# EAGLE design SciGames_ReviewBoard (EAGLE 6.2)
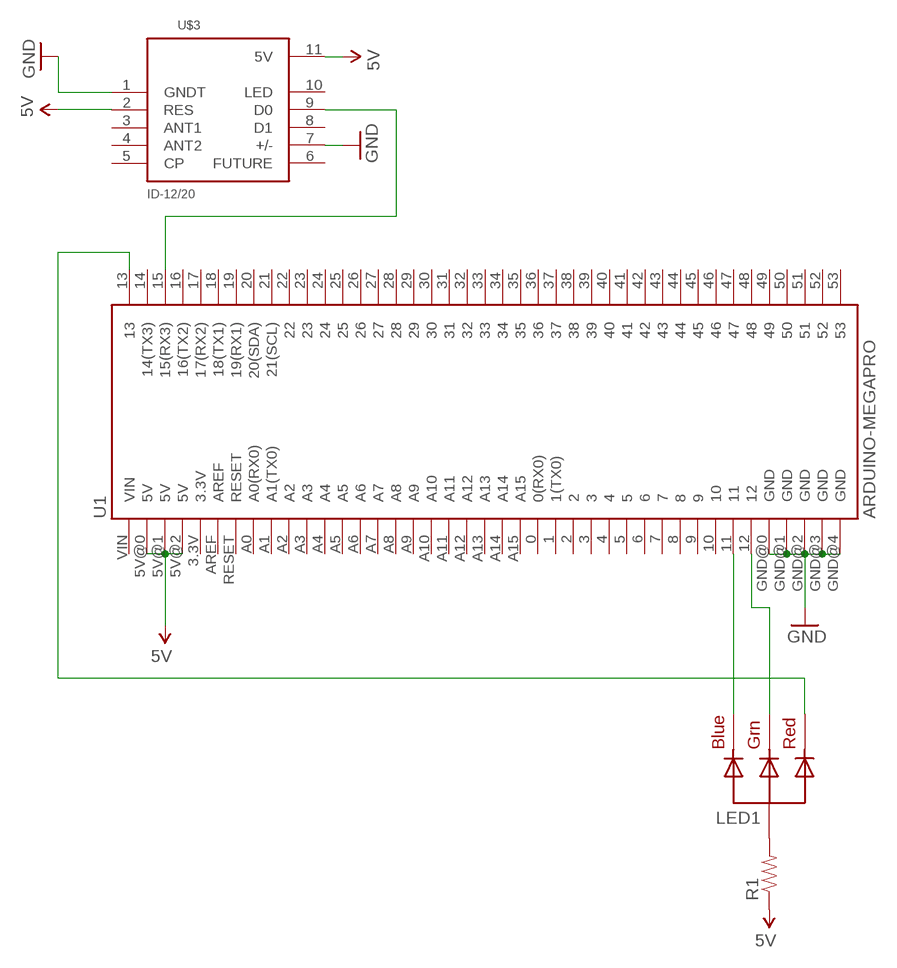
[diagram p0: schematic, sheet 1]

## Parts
LED1  RGBLED_CA-5MM  [LED5MMRGB]
R1  RESISTORPTH-1/6W  [1/6W-RES]
U1  ARDUINO-MEGAPRO  [ARDUINO_MEGA-PRO-3.3V]
U$3  ID-12/20  [ID-12]

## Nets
5V: R1.1 U1.5V@0(5V) U1.5V@1(5V) U1.5V@2(5V) U$3.2(RES) U$3.11(5V)
GND: U1.GND@0(GND) U1.GND@1(GND) U1.GND@2(GND) U1.GND@3(GND) U1.GND@4(GND) U$3.1(GNDT) U$3.7(+/-)
N$1: U1.15(15(RX3)) U$3.9(D0)
N$2: LED1.4(BLUE) U1.11
N$3: LED1.3(GREEN) U1.12
N$4: LED1.1(RED) U1.13
N$5: LED1.2(VCC) R1.2
Unconnected: U1.0(0(RX0)) U1.1(1(TX0)) U1.2 U1.3 U1.3.3V U1.4 U1.5 U1.6 U1.7 U1.8 U1.9 U1.10 U1.14(14(TX3)) U1.16(16(TX2)) U1.17(17(RX2)) U1.18(18(TX1)) U1.19(19(RX1)) U1.20(20(SDA)) U1.21(21(SCL)) U1.22 U1.23 U1.24 U1.25 U1.26 U1.27 U1.28 U1.29 U1.30 U1.31 U1.32 U1.33 U1.34 U1.35 U1.36 U1.37 U1.38 U1.39 U1.40 U1.41 U1.42 U1.43 U1.44 U1.45 U1.46 U1.47 U1.48 U1.49 U1.50 U1.51 U1.52 U1.53 U1.A0(A0(RX0)) U1.A1(A1(TX0)) U1.A2 U1.A3 U1.A4 U1.A5 U1.A6 U1.A7 U1.A8 U1.A9 U1.A10 U1.A11 U1.A12 U1.A13 U1.A14 U1.A15 U1.AREF U1.RESET U1.VIN U$3.3(ANT1) U$3.4(ANT2) U$3.5(CP) U$3.6(FUTURE) U$3.8(D1) U$3.10(LED)

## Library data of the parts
LED1 = adafruit:RGBLED_CA: RGB LED, common-anode 5MM Staggered pins 5mm Piranha package http://www.ladyada.net/library/pcb/eaglelibrary.html
R1 = SparkFun-Passives:RESISTOR: Resistor
U1 = SparkFun:ARDUINO-MEGA: Arduino Mega footprint connections
U$3 = SparkFun-RF:ID-12/20: RFID reader for ID2, ID12, and ID20 Package

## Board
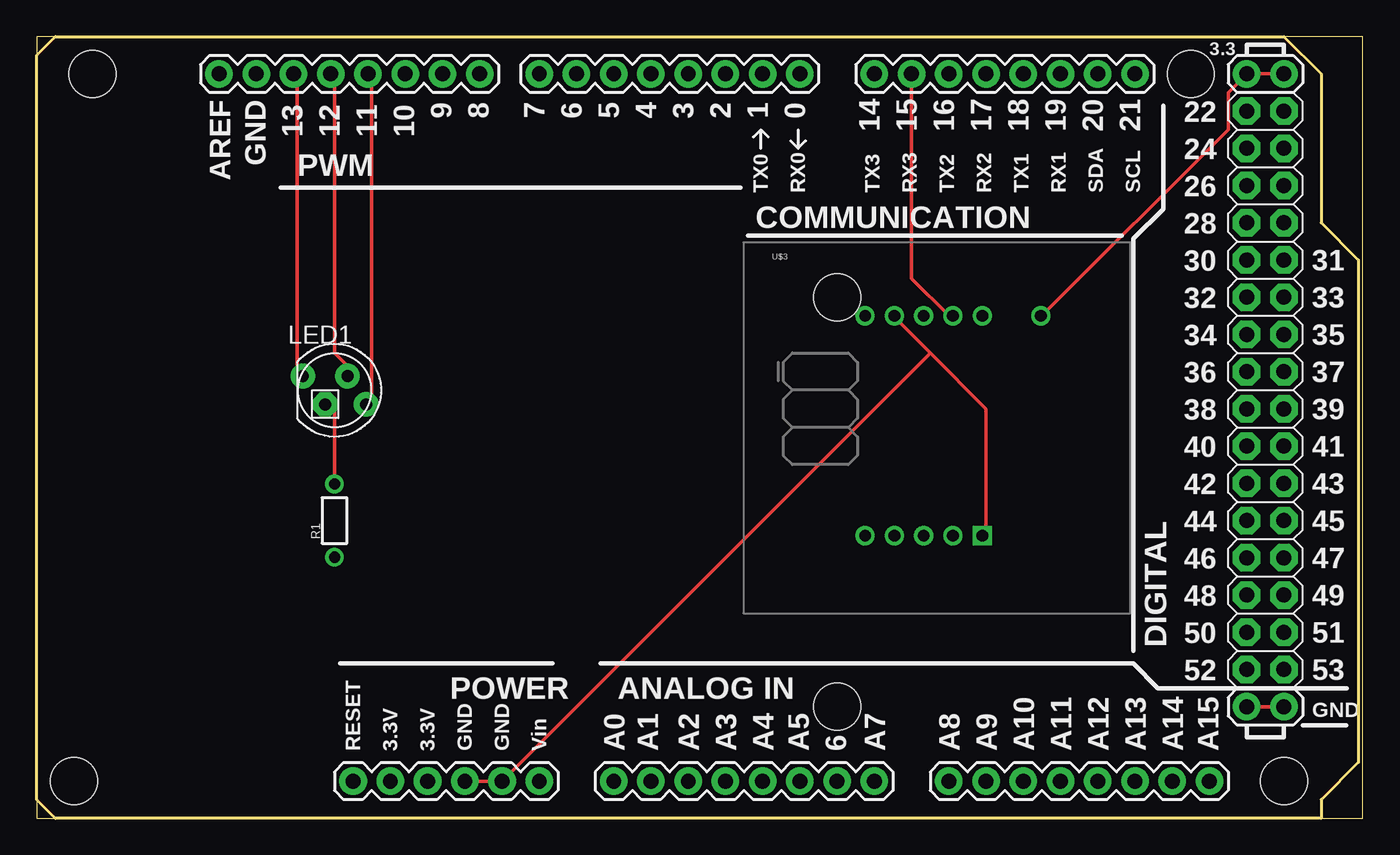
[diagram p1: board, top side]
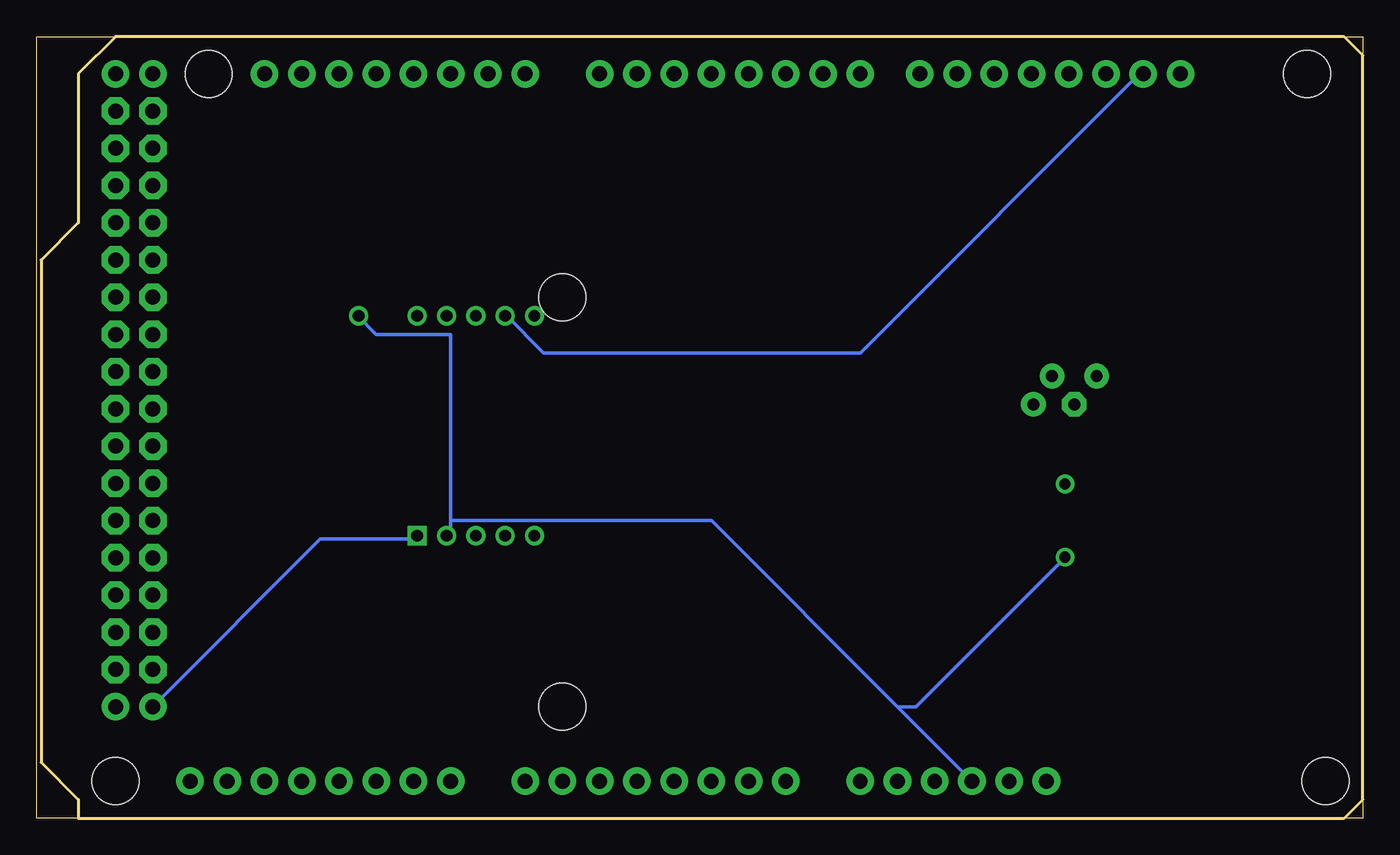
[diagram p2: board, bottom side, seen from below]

Size 90.47 x 53.34 mm. Coordinates in mm from the lower left corner, seen from the top.
Outline: 0,0 90.47,0 90.47,53.33 0,53.33 0,0
Copper layers (1*16): Top 0.035mm / dielectric 1.5mm / Bottom 0.035mm
Design rules: minimum track width 10mil, minimum drill 24mil, track to track 8mil, track to pad 8mil, pad to pad 8mil, via to via 8mil, smd to smd 8mil, copper to edge 40mil, drill to drill 8mil, minimum pad ring 10mil, minimum via ring 8mil, stop-mask expansion 4mil, vias tented up to drill 0mil, thermal gap 10mil

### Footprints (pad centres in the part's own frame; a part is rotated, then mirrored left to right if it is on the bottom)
LED5MMRGB = drill 0.8 pad 1.676: 1 -2.159,0.968; 3 0.889,0.968; 4 2.159,-0.968 | drill 0.8 pad 1.676 octagon: 2 -0.635,-0.968
1/6W-RES = drill 0.762: 1 -2.5,0; 2 2.5,0
ARDUINO_MEGA-PRO-3.3V = drill 1.016 pad 1.88: 0 52.07,50.8; 1 49.53,50.8; 2 46.99,50.8; 3 44.45,50.8; 3.3V 24.13,2.54; 4 41.91,50.8; 5 39.37,50.8; 5V@0 26.67,2.54; 5V@1 82.55,50.8; 5V@2 85.09,50.8; 6 36.83,50.8; 7 34.29,50.8; 8 30.226,50.8; 9 27.686,50.8; 10 25.146,50.8; 11 22.606,50.8; 12 20.066,50.8; 13 17.526,50.8; 14 57.15,50.8; 15 59.69,50.8; 16 62.23,50.8; 17 64.77,50.8; 18 67.31,50.8; 19 69.85,50.8; 20 72.39,50.8; 21 74.93,50.8; A0 39.37,2.54; A1 41.91,2.54; A2 44.45,2.54; A3 46.99,2.54; A4 49.53,2.54; A5 52.07,2.54; A6 54.61,2.54; A7 57.15,2.54; A8 62.23,2.54; A9 64.77,2.54; A10 67.31,2.54; A11 69.85,2.54; A12 72.39,2.54; A13 74.93,2.54; A14 77.47,2.54; A15 80.01,2.54; AREF 12.446,50.8; GND@0 29.21,2.54; GND@1 31.75,2.54; GND@2 82.55,7.62; GND@3 85.09,7.62; GND@4 14.986,50.8; RESET 21.59,2.54; VIN 34.29,2.54 | drill 1.016 pad 1.88 octagon: 22 82.55,48.26; 23 85.09,48.26; 24 82.55,45.72; 25 85.09,45.72; 26 82.55,43.18; 27 85.09,43.18; 28 82.55,40.64; 29 85.09,40.64; 30 82.55,38.1; 31 85.09,38.1; 32 82.55,35.56; 33 85.09,35.56; 34 82.55,33.02; 35 85.09,33.02; 36 82.55,30.48; 37 85.09,30.48; 38 82.55,27.94; 39 85.09,27.94; 40 82.55,25.4; 41 85.09,25.4; 42 82.55,22.86; 43 85.09,22.86; 44 82.55,20.32; 45 85.09,20.32; 46 82.55,17.78; 47 85.09,17.78; 48 82.55,15.24; 49 85.09,15.24; 50 82.55,12.7; 51 85.09,12.7; 52 82.55,10.16; 53 85.09,10.16 | hole 3.2: 3.81,50.8; 2.54,2.54; 54.61,35.56; 54.61,7.62; 78.74,50.8; 85.09,2.54
ID-12 = drill 0.8 square: 1 16.255,5.32 | drill 0.8: 2 14.255,5.32; 3 12.255,5.32; 4 10.255,5.32; 5 8.255,5.32; 6 8.255,20.32; 7 10.255,20.32; 8 12.255,20.32; 9 14.255,20.32; 10 16.255,20.32; 11 20.255,20.32

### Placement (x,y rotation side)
LED1  20.32,29.21 0 top
R1  20.32,20.32 90 top
U1  0,0 0 top
U$3  48.26,13.97 0 top

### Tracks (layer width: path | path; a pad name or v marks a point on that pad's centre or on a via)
5V
  Top 0.254: U1.5V@2 U1.5V@1 81.28,49.53 81.28,46.99 68.58,34.29 U$3.11
  Bottom 0.254: 62.23,20.32 62.23,33.02 67.31,33.02 68.58,34.29 U$3.11 | 62.23,20.32 62.23,19.05 U$3.2 | 31.75,7.62 44.45,20.32 62.23,20.32 | 31.75,7.62 U1.5V@0 | 31.75,7.62 30.48,7.62 20.32,17.78 R1.1
GND
  Top 0.254: U1.GND@0 U1.GND@1 60.96,31.75 | U1.GND@3 U1.GND@2 | 60.96,31.75 64.77,27.94 64.77,19.05 U$3.1 | 60.96,31.75 58.42,34.29 U$3.7
  Bottom 0.254: U1.GND@4 15.24,50.8 34.29,31.75 55.88,31.75 58.42,34.29 U$3.7 | U1.GND@2 71.12,19.05 64.77,19.05 U$3.1
N$1
  Top 0.254: U1.15 59.69,36.83 62.23,34.29 U$3.9
N$2
  Top 0.254: LED1.4 22.86,27.94 22.86,50.8 U1.11
N$3
  Top 0.254: LED1.3 21.59,30.48 20.32,31.75 20.32,50.8 U1.12
N$4
  Top 0.254: LED1.1 17.78,30.48 17.78,50.8 U1.13
N$5
  Top 0.254: R1.2 20.32,27.94 LED1.2

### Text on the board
tValues: V+ | V - | S+ | S - | SciGames Review Board

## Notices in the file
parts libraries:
SparkFun: Licensing: CC v3.0 Share-Alike You are welcome to use this library for commercial purposes.
